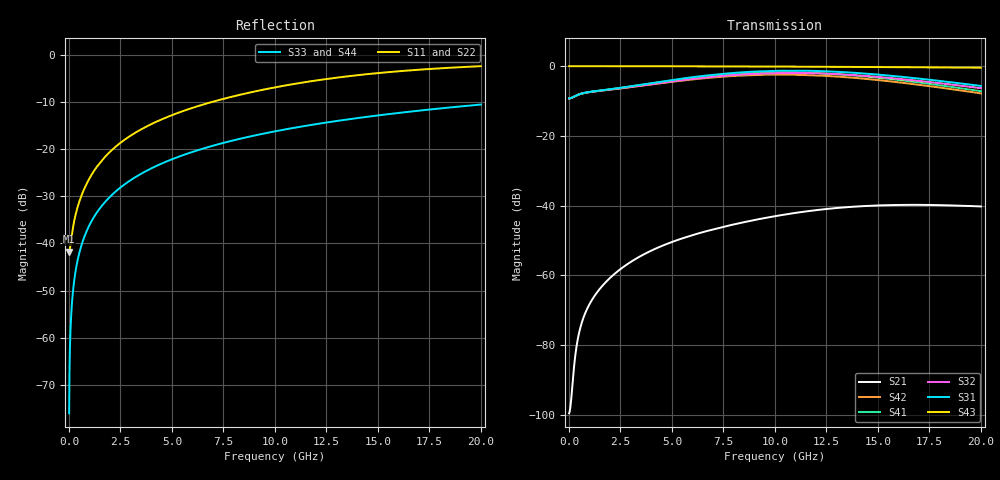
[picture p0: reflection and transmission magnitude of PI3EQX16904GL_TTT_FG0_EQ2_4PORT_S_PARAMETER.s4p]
! NPort=4 DATA=2000 NOISE=0 GROUPDELAY=0 COMPLEX_DATAFORMAT=POLAR
! NumOfBlock=1 NumOfParam=0
! .MODEL Smodel S TSTONEFILE=PI3EQX16904GL_TTT_FG0_EQ2_4PORT_S_PARAMETER.s4p TYPE=S
!  -- The above .MODEL line can be used for the S element in the netlist.
! The s parameter is extracted from the linear redriver, it is not bi-directional; only s(4,1)s(4,2) and s(3,1)s(3,2)
! should be the insertion loss
!Port definition:
!Port1 = input+
!Port2 = input-
!Port3 = output+
!Port4 = output-
# Hz S MA R  50
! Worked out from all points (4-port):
!   2000 points, 10 MHz to 20 GHz, reference 50 ohm
!   strongest paths, dB at 10 MHz, 5.01 GHz, 10.01 GHz, 15.01 GHz, 20 GHz:
!     S43: 0.0, 0.0, -0.1, -0.3, -0.4
!     S31: -9.2, -4.0, -1.3, -2.4, -5.7
!     S32: -9.2, -4.4, -2.0, -3.1, -6.3
!     S41: -9.2, -4.1, -1.8, -3.3, -7.2
!     S42: -9.2, -4.5, -2.4, -4.0, -7.8
!     S21: -99.6, -50.4, -43.0, -39.9, -40.2
!   lowest |S11| = -41.7 dB at 10 MHz (marker M1), VSWR 1.02, Z = 49.2 - j0.0603 ohm
!   |S11| at or under -10 dB: start of sweep to 6.906 GHz
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1e7  0.008182 -175.7  1.05e-05 7.6  0 0.0  0 0.0
     1.05e-05 7.6  0.008182 -175.7  0 0.0  0 0.0
     0.3452 0.2  0.3452 -179.8  0.0001571 -90.0  1 -0.0
     0.3452 -179.8  0.3452 0.2  1 -0.0  0.0001571 -90.0
2e8  0.01483 -130.6  3.383e-05 105.8  0 0.0  0 0.0
     3.383e-05 105.8  0.01483 -130.6  0 0.0  0 0.0
     0.3596 4.4  0.3594 -175.8  0.003142 -90.2  1 -0.2
     0.3596 -175.9  0.3594 3.9  1 -0.2  0.003142 -90.2
6.2e8  0.03268 -112.4  0.0002073 113.7  0 0.0  0 0.0
       0.0002073 113.7  0.03268 -112.4  0 0.0  0 0.0
       0.4054 4.4  0.4045 -176.2  0.009738 -90.6  0.9999 -0.6
       0.4053 -176.7  0.4044 2.7  0.9999 -0.6  0.009738 -90.6
2.97e9  0.1383 -101.6  0.001536 96.2  0 0.0  0 0.0
        0.001536 96.1  0.1384 -101.6  0 0.0  0 0.0
        0.5124 -10.2  0.5014 167.7  0.0466 -92.8  0.9988 -2.7
        0.5101 164.5  0.4991 -17.6  0.9988 -2.7  0.0466 -92.8
1.032e10  0.4681 -113.8  0.007389 42.9  0 0.0  0 0.0
          0.007312 43.2  0.4671 -113.8  0 0.0  0 0.0
          0.8604 -99.7  0.7979 79.2  0.1598 -99.6  0.9861 -9.2
          0.8169 62.4  0.7576 -118.8  0.9861 -9.2  0.1598 -99.6
1.459e10  0.6313 -124.1  0.01003 6.2  0 0.0  0 0.0
          0.009939 7.0  0.6295 -124.1  0 0.0  0 0.0
          0.7745 -161.8  0.7172 17.9  0.2229 -103.4  0.9728 -12.9
          0.7016 -6.3  0.6497 173.4  0.9728 -12.9  0.2229 -103.4
2e10  0.7631 -135.7  0.009764 -34.2  0 0.0  0 0.0
      0.009728 -33.0  0.762 -135.6  0 0.0  0 0.0
      0.5204 129.3  0.4834 -50.4  0.2986 -108.1  0.9506 -17.4
      0.4382 -82.7  0.407 97.6  0.9506 -17.4  0.2986 -108.1
